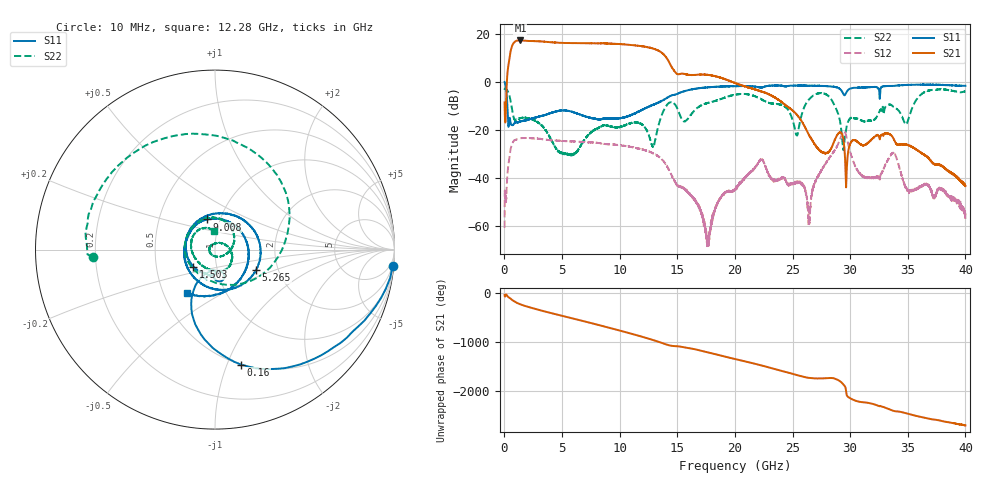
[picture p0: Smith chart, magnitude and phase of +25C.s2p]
!Agilent Technologies,E8363C,MY49030334,A.09.42.15
!Agilent E8363C: A.09.42.15
!Date: Thursday, February 26, 2026 09:20:01
!Correction: S11(Full 2 Port(1,2))
!S21(Full 2 Port(1,2))
!S12(Full 2 Port(1,2))
!S22(Full 2 Port(1,2))
!S2P File: Measurements: S11, S21, S12, S22:
# Hz S  dB  R 50
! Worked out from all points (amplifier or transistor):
!   6401 points, 10 MHz to 40 GHz, reference 50 ohm
!   highest |S21| = 17.2 dB at 1.385 GHz (marker M1)
!   |S21| within 3 dB of that: 610.6 MHz to 12.61 GHz (11.99 GHz wide, 182 % of centre)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
!   unconditionally stable (mu >= 1): start of sweep to end of sweep
!   at 6.671 GHz: K = 1.50, MAG = 16.3 dB, |S12| = -24.9 dB
!   at 20 GHz: K = 20.63, MAG = 5.9 dB, |S12| = -44.5 dB
!   at 40 GHz: K = 9216.71, MAG = -35.8 dB, |S12| = -56.9 dB
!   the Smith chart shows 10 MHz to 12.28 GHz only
!   S11 on the Smith chart (normalised r, x): 10 MHz: 1, -21; 160 MHz: 0.50, -1.12; 1.503 GHz: 0.77, -0.15; 5.265 GHz: 1.53, -0.38; 9.008 GHz: 0.86, +0.30; 12.28 GHz: 0.66, -0.35
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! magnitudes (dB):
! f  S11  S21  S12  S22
! 10 MHz  0.0  -8.5  -60.6  -3.3
! 160 MHz  -3.7  -5.2  -48.6  -3.0
! 622.3 MHz  -17.8  14.4  -26.3  -10.4
! 1.385 GHz  -16.5  17.2  -23.4  -15.1
! 1.503 GHz  -16.3  17.2  -23.3  -15.0
! 5.265 GHz  -11.8  16.2  -24.6  -29.9
! 6.677 GHz  -13.8  16.1  -24.9  -25.9
! 9.008 GHz  -15.2  15.9  -25.9  -18.2
! 12.28 GHz  -10.8  14.6  -28.5  -19.6
! 13.34 GHz  -8.6  13.0  -30.9  -18.5
! 17.63 GHz  -2.3  2.9  -66.6  -8.8
! 20 GHz  -1.8  -0.4  -44.5  -5.3
! 22.27 GHz  -2.4  -4.0  -32.1  -7.2
! 25.35 GHz  -1.5  -13.6  -41.8  -22.1
! 26.67 GHz  -1.6  -24.0  -46.6  -6.1
! 28.3 GHz  -1.9  -28.0  -30.7  -6.9
! 29.42 GHz  -5.1  -23.9  -20.6  -28.0
! 31.15 GHz  -2.3  -26.3  -39.4  -16.4
! 33.34 GHz  -1.7  -21.6  -31.9  -9.3
! 34.84 GHz  -1.3  -26.0  -43.9  -17.6
! 36.49 GHz  -1.2  -30.4  -42.9  -4.1
! 40 GHz  -1.6  -43.2  -56.9  -3.9
